
//840D





//SIN_SL


ORGANIZATION_BLOCK OB 1

      VERSION: 1.0
VAR_TEMP

      OB1_EV_CLASS : BYTE;
      OB1_SCAN_1 : BYTE;
      OB1_PRIORITY : BYTE;
      OB1_OB_NUMBR : BYTE;
      OB1_RESERVED_1 : BYTE;
      OB1_RESERVED_2 : BYTE;
      OB1_PREV_CYCLE : INT;
      OB1_MIN_CYCLE : INT;
      OB1_MAX_CYCLE : INT;
      OB1_DATE_TIME : DATE_AND_TIME;
END_VAR

BEGIN

      CALL FC 2;

      //Insert User program from here


END_ORGANIZATION_BLOCK


//*************************************************************
ORGANIZATION_BLOCK OB 100

      VERSION: 1.0


VAR_TEMP
      OB100_EV_CLASS : BYTE;
      OB100_STRTUP : BYTE;
      OB100_PRIORITY : BYTE;
      OB100_OB_NUMBR : BYTE;
      OB100_RESERVED_1 : BYTE;
      OB100_RESERVED_2 : BYTE;
      OB100_STOP : WORD;
      OB100_RESERVED_3 : WORD;
      OB100_RESERVED_4 : WORD;
      OB100_DATE_TIME : DATE_AND_TIME;
END_VAR

BEGIN
Call fb 1, db 7(
      MCPNum :=1,
      MCP1In :=P#E0.0,
      MCP1Out        :=P#A0.0,
      MCP1StatSend   :=P#A8.0,
      MCP1StatRec    :=P#A12.0,
      MCP1BusAdr     :=6);

      //Insert User program from here


END_ORGANIZATION_BLOCK

//*************************************************************
ORGANIZATION_BLOCK OB 40

      VERSION: 1.0
VAR_TEMP

      OB40_EV_CLASS : BYTE;
      OB40_STRT_INF : BYTE;
      OB40_PRIORITY : BYTE;
      OB40_OB_NUMBR : BYTE;
      OB40_RESERVED_1 : BYTE;
      OB40_MDL_ID : BYTE;
      OB40_MDL_ADDR : INT;
      OB40_POINT_ADDR : DWORD;
      OB40_DATE_TIME : DATE_AND_TIME;

//data for the Basic program
      GP_IRFromNCK : BOOL;          //Interrupt from NCK
      GP_TM : BOOL;                 //Toolmanagment
      GP_InPosition : ARRAY [1..31] OF BOOL;  //InPos Signal from FC15,16,18
      GP_AuxFunction : ARRAY [1..10] OF BOOL;   //auxiliary functions
      GP_FMBlock : ARRAY [1..10] OF BOOL; //not used

//Insert User-data from here

END_VAR

BEGIN

      CALL FC 3;

      //Insert User program from here


END_ORGANIZATION_BLOCK

//*************************************************************
ORGANIZATION_BLOCK OB 82
TITLE = "I/O Point Fault"
VERSION : 1.0


VAR_TEMP
  OB82_EV_CLASS : BYTE ;    //16#39, Event class 3, Entering event state, Internal fault event
  OB82_FLT_ID : BYTE ;  //16#XX, Fault identifcation code
  OB82_PRIORITY : BYTE ;    //Priority of OB Execution
  OB82_OB_NUMBR : BYTE ;    //82 (Organization block 82, OB82)
  OB82_RESERVED_1 : BYTE ;  //Reserved for system
  OB82_IO_FLAG : BYTE ; //Input (01010100), Output (01010101)
  OB82_MDL_ADDR : WORD ;    //Base address of module with fault
  OB82_MDL_DEFECT : BOOL ;  //Module defective
  OB82_INT_FAULT : BOOL ;   //Internal fault
  OB82_EXT_FAULT : BOOL ;   //External fault
  OB82_PNT_INFO : BOOL ;    //Point information
  OB82_EXT_VOLTAGE : BOOL ; //External voltage low
  OB82_FLD_CONNCTR : BOOL ; //Field wiring connector missing
  OB82_NO_CONFIG : BOOL ;   //Module has no configuration data
  OB82_CONFIG_ERR : BOOL ;  //Module has configuration error
  OB82_MDL_TYPE : BYTE ;    //Type of module
  OB82_SUB_MDL_ERR : BOOL ; //Sub-Module is missing or has error
  OB82_COMM_FAULT : BOOL ;  //Communication fault
  OB82_MDL_STOP : BOOL ;    //Module is stopped
  OB82_WTCH_DOG_FLT : BOOL ;    //Watch dog timer stopped module
  OB82_INT_PS_FLT : BOOL ;  //Internal power supply fault
  OB82_PRIM_BATT_FLT : BOOL ;   //Primary battery is in fault
  OB82_BCKUP_BATT_FLT : BOOL ;  //Backup battery is in fault
  OB82_RESERVED_2 : BOOL ;  //Reserved for system
  OB82_RACK_FLT : BOOL ;    //Rack fault, only for bus interface module
  OB82_PROC_FLT : BOOL ;    //Processor fault
  OB82_EPROM_FLT : BOOL ;   //EPROM fault
  OB82_RAM_FLT : BOOL ; //RAM fault
  OB82_ADU_FLT : BOOL ; //ADU fault
  OB82_FUSE_FLT : BOOL ;    //Fuse fault
  OB82_HW_INTR_FLT : BOOL ; //Hardware interupt input in fault
  OB82_RESERVED_3 : BOOL ;  //Reserved for system
  OB82_DATE_TIME : DATE_AND_TIME ;  //Date and time OB82 started
END_VAR
BEGIN
NETWORK
TITLE =Detailed Diagnosis in OB82 (interrupt)

      CALL FC     5 (
           PlcStop                  := TRUE);


END_ORGANIZATION_BLOCK

//*************************************************************
ORGANIZATION_BLOCK OB 86
TITLE = "Loss Of Rack Fault"
VERSION : 1.0


VAR_TEMP
  OB86_EV_CLASS : BYTE ;    //16#38/39 Event class 3
  OB86_FLT_ID : BYTE ;  //16#C1/C4/C5, Fault identifcation code
  OB86_PRIORITY : BYTE ;    //Priority of OB Execution
  OB86_OB_NUMBR : BYTE ;    //86 (Organization block 86, OB86)
  OB86_RESERVED_1 : BYTE ;  //Reserved for system
  OB86_RESERVED_2 : BYTE ;  //Reserved for system
  OB86_MDL_ADDR : WORD ;    //Base address of IM module in rack with fault
  OB86_RACKS_FLTD : ARRAY  [0 .. 31 ] OF BOOL ; //Racks in fault
  OB86_DATE_TIME : DATE_AND_TIME ;  //Date and time OB86 started
END_VAR
BEGIN
NETWORK
TITLE =Detailed Diagnosis in OB86 (interrupt)

      CALL FC     5 (
           PlcStop                  := TRUE);


END_ORGANIZATION_BLOCK

